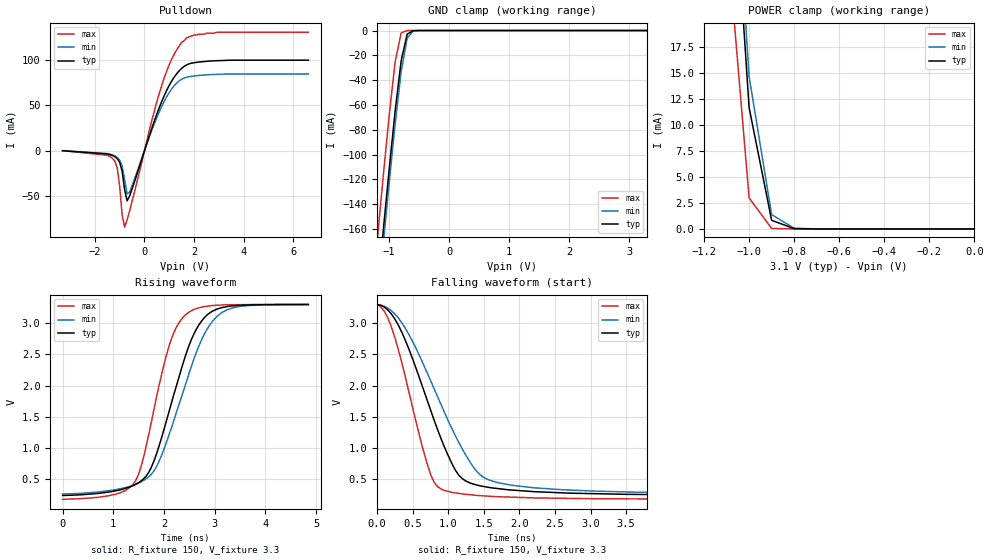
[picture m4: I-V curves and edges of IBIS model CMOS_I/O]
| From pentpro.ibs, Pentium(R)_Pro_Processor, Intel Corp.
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[Model]   CMOS_I/O
Model_type  I/O_open_drain
Polarity   Inverting
Enable   Active-Low
Vinl = 0.8
Vinh = 2.0
Vmeas = 1.50
Cref  = 0.00p
Rref  = 150.00
Vref  = 3.30
|Variable   typ   min   max
C_comp   2.6p   2.3p   2.8p
|Variable   typ   min   max
[Voltage range] 3.1   2.845  3.255
|Variable   typ   min   max
[Temperature Range] 80   0   100
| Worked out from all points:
|   slope of the pulldown table from 0 to 0.465 V, typ, clamps not added: 12.3 ohm
|   GND clamp passes 1 mA (typ) near -0.63 V on its own axis
|   POWER clamp passes 1 mA (typ) near -0.90 V on its own axis
|   rising waveform, R_fixture 150, V_fixture 3.3: 20-80 % time 688ps typ, 773ps min, 536ps max; typ from 0.243 V to 3.3 V
|   falling waveform, R_fixture 150, V_fixture 3.3: 20-80 % time 600ps typ, 749ps min, 417ps max; typ from 3.3 V to 0.243 V
[Pulldown]
|Volts   typ   min   max
-3.3V     0A         0A         0A
-1.2V     -6.46mA    -5.59mA    -11.3mA
-1V       -12.8mA    -10.3mA    -39.2mA
-900mV    -22.6mA    -16.8mA    -70.8mA
-800mV    -43mA      -31.8mA    -84mA
-700mV    -55.1mA    -47.4mA    -76.1mA
-600mV    -49.9mA    -45.5mA    -66.1mA
600mV     47.6mA     43mA       63.3mA
1.1V      76.7mA     68mA       101mA
1.5V      90.5mA     78.5mA     119mA
2.9V      98.8mA     83.8mA     130mA
6.6V      99.4mA     84.3mA     130mA
[Pullup]
|Volts   typ   min   max
-3.3V     0A         0A         0A
6.6V      0A         0A         0A
[GND_clamp]
|Volts   typ   min   max
-3.3V     -1.36A     -1.38A     -1.3A
-1.2V     -214mA     -225mA     -170mA
-1.1V     -162mA     -173mA     -118mA
-1V       -112mA     -123mA     -68.7mA
-900mV    -64.5mA    -75.2mA    -25.1mA
-800mV    -24.3mA    -33.1mA    -1.87mA
-700mV    -2.93mA    -6.13mA    -28.1uA
-600mV    -120uA     -353uA     0A
3.3V      0A         0A         0A
[POWER_clamp]
|Volts   typ   min   max
-3.3V     1.19A      1.21A      1.19A
-1.1V     44.5mA     48.7mA     28.8mA
-1V       11.7mA     14.7mA     2.99mA
-900mV    835uA      1.39mA     53.6uA
-800mV    32.8uA     66.7uA     0A
0V        0A         0A         0A
[Ramp]
|Variable   typ   min   max
dV/dt_r   1.84/0.65n 1.82/0.75n 1.87/0.53n
dV/dt_f   1.84/0.60n 1.82/0.75n 1.87/0.39n
[Rising Waveform]
R_fixture = 150
V_fixture = 3.3
C_fixture = 0.00pF
|Time   Typ(v)   Min(v)   Max(v)
0s        243mV      267mV      182mV
950ps     303mV      NA         NA
1.4ns     404mV      NA         431mV
1.55ns    477mV      461mV      709mV
1.8ns     789mV      634mV      NA
2.2ns     1.872V     NA         2.857V
2.45ns    2.54V      NA         3.151V
2.8ns     3.091V     2.83V      3.267V
3.15ns    3.252V     3.174V     NA
4.85ns    3.3V       3.3V       3.3V
[Falling Waveform]
R_fixture = 150
V_fixture = 3.3
C_fixture = 0.00pF
|Time   Typ(v)   Min(v)   Max(v)
0s        3.3V       3.3V       3.3V
150ps     3.213V     3.242V     3.084V
350ps     2.848V     3.002V     2.351V
650ps     1.943V     NA         961mV
800ps     1.452V     NA         457mV
950ps     1.008V     1.563V     323mV
1.15ns    566mV      1.086V     NA
1.45ns    397mV      573mV      NA
1.85ns    334mV      NA         NA
7.8ns     243mV      268mV      182mV
